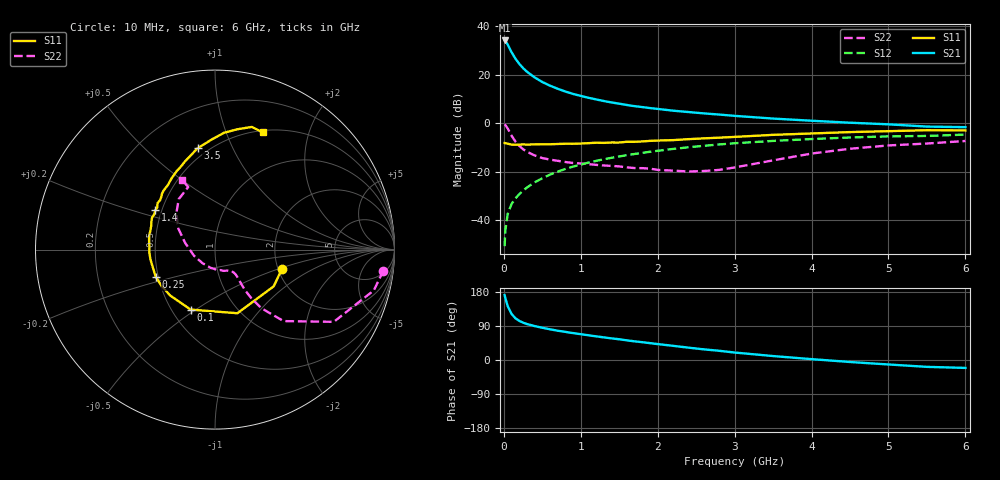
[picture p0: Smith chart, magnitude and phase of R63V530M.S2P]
! SIEMENS Small Signal Semiconductors
! BFR193
! Si NPN RF Bipolar Junction Transistor in SOT23
! VCE = 3.5 V  IC = 30 mA
! Common Emitter S-Parameters:  May  1996
# GHz  S  MA  R  50
!  f  S11  S21  S12  S22
! GHz  MAG  ANG  MAG  ANG  MAG  ANG  MAG  ANG
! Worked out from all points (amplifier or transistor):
!   36 points, 10 MHz to 6 GHz, reference 50 ohm
!   highest |S21| = 34.1 dB at 10 MHz (marker M1)
!   |S21| within 3 dB of that: start of sweep to 70.91 MHz
!   unconditionally stable (mu >= 1): 473.3 MHz to 1.912 GHz
!   at 250 MHz: K = 0.90, MSG = 25.3 dB, |S12| = -27.9 dB
!   at 1.4 GHz: K = 1.02, MAG = 10.5 dB, |S12| = -14.3 dB
!   at 6 GHz: K = 0.94, MSG = 1.5 dB, |S12| = -4.7 dB
!   lowest NFmin = 1.90 dB at 450 MHz
!   S11 on the Smith chart (normalised r, x): 10 MHz: 2.10, -0.53; 100 MHz: 0.62, -0.48; 250 MHz: 0.48, -0.17; 1.4 GHz: 0.46, +0.24; 3.5 GHz: 0.44, +0.74; 6 GHz: 0.52, +1.35
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0.01  0.3881 -16.1  50.6 171.2  0.0029 81.6  0.9456 -7.1
0.02  0.3859 -32.0  49.36 162.8  0.0062 78.6  0.9136 -14.4
0.05  0.3759 -70.6  41.63 142.4  0.0134 71.0  0.7747 -31.3
0.1  0.3608 -112.1  29.07 121.8  0.0215 65.3  0.5519 -46.2
0.15  0.3574 -134.3  21.42 110.2  0.028 65.9  0.4174 -51.6
0.2  0.3601 -146.0  16.72 103.4  0.0342 67.6  0.3402 -53.2
0.25  0.3635 -155.2  13.61 98.5  0.0405 69.0  0.2894 -53.5
0.3  0.3604 -161.7  11.49 95.0  0.0469 70.0  0.2567 -53.0
0.4  0.364 -171.5  8.758 89.6  0.06 71.5  0.2156 -51.7
0.5  0.3662 -177.5  7.034 85.1  0.0728 71.8  0.1904 -50.5
0.6  0.3663 176.7  5.916 81.0  0.0865 71.8  0.1767 -50.3
0.7  0.3711 171.9  5.104 77.3  0.0998 71.1  0.1671 -50.6
0.8  0.3752 167.7  4.476 74.2  0.1134 70.2  0.1578 -51.7
0.9  0.3748 163.9  3.998 71.0  0.1268 69.4  0.1504 -52.2
1.1  0.3862 156.7  3.329 65.2  0.1532 67.2  0.1429 -56.4
1.4  0.3983 146.7  2.664 57.1  0.1925 63.4  0.1311 -64.3
1.7  0.4117 137.9  2.236 49.2  0.2308 59.4  0.1183 -74.9
2.2  0.4457 126.0  1.804 37.4  0.2934 52.2  0.1048 -102.6
3.5  0.5726 99.8  1.24 10.4  0.4293 32.1  0.1705 167.4
4.5  0.6528 85.6  1.019 -5.3  0.5053 17.9  0.2958 136.7
5.5  0.7136 73.3  0.848 -18.1  0.5435 3.9  0.379 113.2
6  0.7053 67.8  0.825 -20.9  0.5795 -0.2  0.4282 115.2
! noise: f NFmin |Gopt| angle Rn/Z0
0.45  1.9  0.4  180  0.09
0.9  1.95  0.43  -173  0.11
1.8  2.4  0.58  -144  0.24
